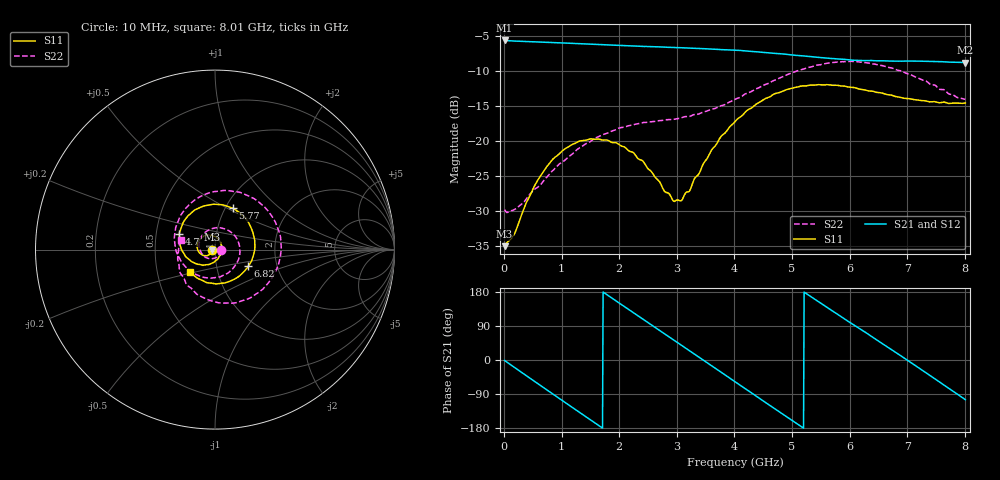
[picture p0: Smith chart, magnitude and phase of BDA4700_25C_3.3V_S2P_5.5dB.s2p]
!Agilent Technologies,E5071B,MY42404982,A.09.10
!Date: Mon Oct 20 18:05:18 2025
!Data & Calibration Information:
!Freq	S11:SOLT2(ON)	S21:SOLT2(ON)	S12:SOLT2(ON)	S22:SOLT2(ON)
# Hz S RI R 50
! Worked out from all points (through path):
!   801 points, 10 MHz to 8.01 GHz, reference 50 ohm
!   highest |S21| = -5.62 dB at 10 MHz (marker M1); lowest = -8.8 dB at 8.01 GHz (marker M2)
!   group delay of S21, straight-line fit = 285 ps
!   lowest |S11| = -35.0 dB at 10 MHz (marker M3), VSWR 1.04, Z = 48.3 - j0.107 ohm
!   |S11| at or under -10 dB: start of sweep to end of sweep
!   |S22| runs from -30.2 to -8.6 dB; largest |S21 - S12| = 0.006
!   S11 on the Smith chart (normalised r, x): 10 MHz: 0.97, -0.00; 4.7 GHz: 0.66, +0.12; 5.77 GHz: 1.08, +0.53; 6.82 GHz: 1.42, -0.28; 8.01 GHz: 0.74, -0.19
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1e7  -0.0177 -0.00111  0.5235 -0.0112  0.5233 -0.0117  0.0323 -0.00257
3.3e8  -0.0238 -0.0208  0.4205 -0.2984  0.4202 -0.2984  0.0224 -0.0283
7.1e8  -0.0525 -0.0343  0.1287 -0.4919  0.1285 -0.4921  -0.0163 -0.0509
1.02e9  -0.0829 -0.0217  -0.1538 -0.4783  -0.1539 -0.4786  -0.0615 -0.0359
1.35e9  -0.0998 0.0133  -0.3921 -0.3036  -0.3922 -0.3037  -0.0885 0.0225
1.64e9  -0.0904 0.0501  -0.486 -0.0645  -0.4862 -0.0645  -0.0674 0.0837
1.93e9  -0.0609 0.0759  -0.4471 0.1855  -0.4471 0.1857  -0.00256 0.1201
2.32e9  -0.00895 0.0747  -0.2182 0.4239  -0.218 0.4241  0.0977 0.0901
2.68e9  0.0291 0.0434  0.0808 0.4639  0.0799 0.464  0.1395 -0.00809
3.05e9  0.036 -0.0106  0.3463 0.3097  0.3431 0.3123  0.094 -0.111
3.37e9  0.0101 -0.0565  0.4533 0.0723  0.4536 0.0721  0.00358 -0.1556
4.01e9  -0.1159 -0.0742  0.2414 -0.3749  0.242 -0.3743  -0.1861 -0.0695
4.36e9  -0.1805 -0.0102  -0.0259 -0.4344  -0.0266 -0.4353  -0.2267 0.0595
4.7e9  -0.1987 0.0895  -0.2651 -0.3303  -0.2637 -0.3315  -0.1853 0.2
5.03e9  -0.1514 0.1871  -0.3919 -0.1243  -0.393 -0.1242  -0.0637 0.3043
5.35e9  -0.0544 0.2451  -0.3865 0.1049  -0.387 0.1027  0.1031 0.3242
5.77e9  0.0984 0.2303  -0.209 0.3256  -0.208 0.3259  0.3029 0.2059
6.2e9  0.2034 0.1159  0.0642 0.3704  0.0694 0.3709  0.3647 -0.0335
6.68e9  0.208 -0.0504  0.3166 0.1979  0.3174 0.1968  0.2195 -0.2539
6.82e9  0.1852 -0.0929  0.3544 0.115  0.3552 0.1125  0.151 -0.2849
7.31e9  0.0581 -0.185  0.3148 -0.1979  0.315 -0.1984  -0.0953 -0.2526
8.01e9  -0.1381 -0.1262  -0.0935 -0.3519  -0.0926 -0.3523  -0.1921 0.0508
